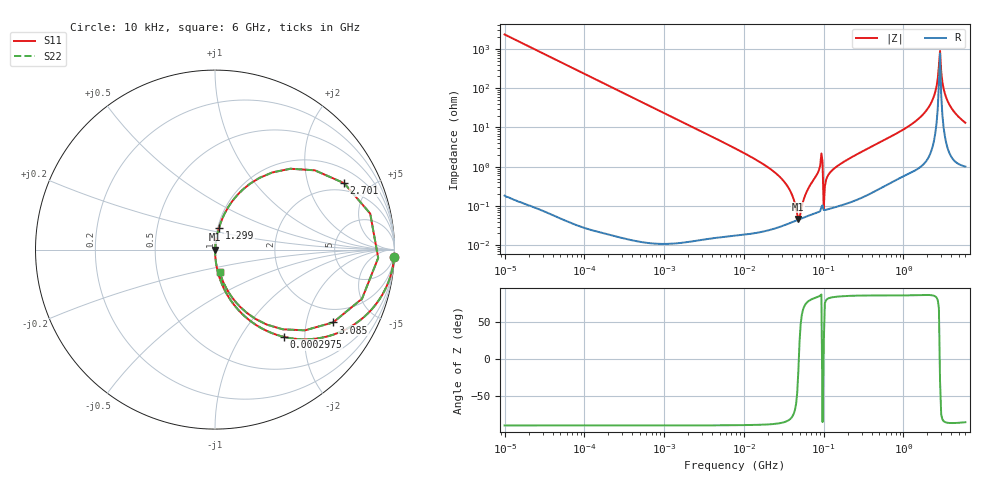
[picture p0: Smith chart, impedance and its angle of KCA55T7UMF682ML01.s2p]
!Murata Part Number: KCA55T7UMF682ML01
!These Parameters are Measured in Series Mode Connection
!Data Generated on Jan 08, 2026
!  o--ll--o
!Port1  Port2
!  o------o
!Operation Temp=25[degC], DC Bias Voltage=0[V]
!Freq. Start=10[kHz] Stop=6[GHz] 401[Steps]
# Hz S RI R 50
!Freq.(Hz) S11(Real) S11(Imag) S21(Real) S21(Imag) S12(Real) S12(Imag) S22(Real) S22(Imag)
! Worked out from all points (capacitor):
!   401 points, 10 kHz to 6 GHz, reference 50 ohm
!   read as one part in series: C = 6.79 nF near 10.69 kHz
!   lowest |Z| = 46.5 mohm at 48.26 MHz (marker M1)
!   series resonance near 48.91 MHz, so ESL is about 1.6 nH
!   S11 on the Smith chart (normalised r, x): 10 kHz: 1, -47; 297.5 kHz: 1.00, -1.58; 1.299 GHz: 1.01, +0.25; 2.701 GHz: 1.60, +3.43; 3.085 GHz: 1.43, -2.88; 6 GHz: 1.02, -0.26
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10000  0.9982 -0.0426  0.00182 0.0426  0.00182 0.0426  0.9982 -0.0426
92862  0.8642 -0.3425  0.1358 0.3425  0.1358 0.3425  0.8642 -0.3425
297460  0.383 -0.486  0.617 0.486  0.617 0.486  0.383 -0.486
862344  0.0688 -0.2529  0.9312 0.2529  0.9312 0.2529  0.0688 -0.2529
7745967  0.00104 -0.0294  0.999 0.0294  0.999 0.0294  0.00104 -0.0294
2.930156e7  0.000327 -0.0051  0.9997 0.0051  0.9997 0.0051  0.000327 -0.0051
3.823436e7  0.000375 -0.00237  0.9996 0.00237  0.9996 0.00237  0.000375 -0.00237
4.825823e7  0.000447 -0.000128  0.9996 0.000128  0.9996 0.000128  0.000447 -0.000128
7.193098e7  0.000628 0.00405  0.9994 -0.00405  0.9994 -0.00405  0.000628 0.00405
9.078908e7  0.000861 0.0109  0.9991 -0.0109  0.9991 -0.0109  0.000861 0.0109
1.072162e8  0.00082 0.00447  0.9992 -0.00447  0.9992 -0.00447  0.00082 0.00447
1.145912e8  0.000867 0.00614  0.9991 -0.00614  0.9991 -0.00614  0.000867 0.00614
1.446335e8  0.00105 0.00991  0.999 -0.00991  0.999 -0.00991  0.00105 0.00991
6.67969e8  0.00681 0.0553  0.9932 -0.0553  0.9932 -0.0553  0.00681 0.0553
1.299164e9  0.0224 0.1215  0.9776 -0.1215  0.9776 -0.1215  0.0224 0.1215
2.139659e9  0.1289 0.3087  0.8711 -0.3087  0.8711 -0.3087  0.1289 0.3087
2.526803e9  0.4203 0.4505  0.5797 -0.4505  0.5797 -0.4505  0.4203 0.4505
2.700612e9  0.7196 0.37  0.2804 -0.37  0.2804 -0.37  0.7196 0.37
3.084918e9  0.6581 -0.4059  0.3419 0.4059  0.3419 0.4059  0.6581 -0.4059
3.297118e9  0.3778 -0.4442  0.6222 0.4442  0.6222 0.4442  0.3778 -0.4442
3.766309e9  0.144 -0.3229  0.856 0.3229  0.856 0.3229  0.144 -0.3229
6e9  0.0265 -0.1266  0.9735 0.1266  0.9735 0.1266  0.0265 -0.1266
